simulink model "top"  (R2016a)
settings: Solver=FixedStepAuto  StartTime=0.0  StopTime=0.1  RelTol=1e-3
PreLoadFcn:
  | % ---  DO NOT REMOVE THIS CODE (2025.1)   ---
  |     % create Simulink variants
  |     if not(exist('variant_simulation', 'var'))
  |         variant_simulation = Simulink.Variant('SIMULINK_MODE==0');
  |     end
  |     if not(exist('variant_generation', 'var'))
  |         variant_generation = Simulink.Variant('SIMULINK_MODE==1');
  |     end
  | 
  |     % check SDK version
  |     required_lib_version = 3900.3;
  |     required_lib_ver_str = '2025.1';
  |     lib_path = [getenv('IX_SIMULINK_ACG_BB_3') '\simulink\blocks\BoomBox.slx'];
  |     if exist(lib_path, 'file')
  |         lib_version = str2double(Simulink.MDLInfo(lib_path).ModelVersion); % fullpath to avoid getting shadowing files
  |         if lib_version < required_lib_version || isnan(lib_version)
  |             error(['The model ''' bdroot ''' has been saved with a more recent version of ACG SDK (' required_lib_ver_str ') and might not work as expected. <a href="matlab:private_end_string = ''--- PLACE YOUR CODE BELOW THIS LINE ---'';private_fcn = get_param(bdroot, ''PreLoadFcn'');private_end_index = strfind(private_fcn, private_end_string);set_param(bdroot, ''PreLoadFcn'', strtrim(private_fcn(private_end_index(end)+length(private_end_string):end)));private_fcn = get_param(bdroot, ''PostLoadFcn'');private_end_index = strfind(private_fcn, private_end_string);set_param(bdroot, ''PostLoadFcn'', strtrim(private_fcn(private_end_index(end)+length(private_end_string):end)));private_fcn = get_param(bdroot, ''InitFcn'');private_end_index = strfind(private_fcn, private_end_string);set_param(bdroot, ''InitFcn'', strtrim(private_fcn(private_end_index(end)+length(private_end_string):end)));clear private_end_string private_fcn private_end_index;open(bdroot);">Click here</a> to continue anyway, or download the latest version of the SDK at <a href="www.imperix.com/downloads">www.imperix.ch/downloads</a>.']);
  |         end
  |     elseif exist(getenv('IX_SIMULINK_ACG_BB_3'), 'dir')
  |         error(['Library file for imperix ACG SDK not found in path ''' lib_path '''. Please try to re-install ACG SDK (<a href="www.imperix.com/downloads">www.imperix.ch/downloads</a>).']);
  |     else
  |         error('ACG SDK is not installed on this computer and the model will not work as expected. Please download ACG SDK at <a href="www.imperix.com/downloads">www.imperix.ch/downloads</a>, install it, and reopen the model.');
  |     end
  |     clear required_lib_version required_lib_ver_str lib_path lib_version;
  | 
  |     ix_acg_path = getenv('IX_SIMULINK_ACG_BB_3');
  |     addpath(fullfile(ix_acg_path, 'simulink\target'));
  |     addpath(fullfile(ix_acg_path, 'simulink\blocks'));
  |     addpath(fullfile(ix_acg_path, 'simulink\functions'));
  |     sl_refresh_customizations;
  |     clear ix_acg_path;
  | 
  |     % The SIMULINK_MODE variable is created in the base
  |     % workspace in the PostLoadFcn from the block whose id is kb0101
  |     % All opened models share a common variant configuration.
  | 
  |     Model_PreLoadFcn(bdroot);
  | % --- PLACE YOUR CODE BELOW THIS LINE ---
PostLoadFcn:
  | % ---  DO NOT REMOVE THIS CODE (2025.1)   ---
  |     % change the execution mode of simulink depending on the radio button:
  |     if(strcmp('Automated Code Generation',get_param(Find_imperix_blocks(bdroot,'Configuration'),'SLMODE')))
  |         assignin('base', 'SIMULINK_MODE', 1);
  |     else
  |         assignin('base', 'SIMULINK_MODE', 0);
  |     end
  | 
  |     Model_PostLoadFcn(bdroot);
  | % --- PLACE YOUR CODE BELOW THIS LINE ---
InitFcn:
  | % ---  DO NOT REMOVE THIS CODE (2025.1)   ---
  |     % check SDK version
  |     required_lib_version = 3900.3;
  |     required_lib_ver_str = '2025.1';
  |     lib_path = [getenv('IX_SIMULINK_ACG_BB_3') '\simulink\blocks\BoomBox.slx'];
  |     if exist(lib_path, 'file')
  |         lib_version = str2double(Simulink.MDLInfo(lib_path).ModelVersion); % fullpath to avoid getting shadowing files
  |         if lib_version < required_lib_version || isnan(lib_version)
  |             error(['The model ''' bdroot ''' has been saved with a more recent version of ACG SDK (' required_lib_ver_str ') and might not work as expected. <a href="matlab:private_end_string = ''--- PLACE YOUR CODE BELOW THIS LINE ---'';private_fcn = get_param(bdroot, ''PreLoadFcn'');private_end_index = strfind(private_fcn, private_end_string);set_param(bdroot, ''PreLoadFcn'', strtrim(private_fcn(private_end_index(end)+length(private_end_string):end)));private_fcn = get_param(bdroot, ''PostLoadFcn'');private_end_index = strfind(private_fcn, private_end_string);set_param(bdroot, ''PostLoadFcn'', strtrim(private_fcn(private_end_index(end)+length(private_end_string):end)));private_fcn = get_param(bdroot, ''InitFcn'');private_end_index = strfind(private_fcn, private_end_string);set_param(bdroot, ''InitFcn'', strtrim(private_fcn(private_end_index(end)+length(private_end_string):end)));clear private_end_string private_fcn private_end_index;open(bdroot);">Click here</a> to continue anyway, or download the latest version of the SDK at <a href="www.imperix.com/downloads">www.imperix.ch/downloads</a>.']);
  |         end
  |     elseif exist(getenv('IX_SIMULINK_ACG_BB_3'), 'dir')
  |         error(['Library file for imperix ACG SDK not found in path ''' lib_path '''. Please try to re-install ACG SDK (<a href="www.imperix.com/downloads">www.imperix.ch/downloads</a>).']);
  |     else
  |         error('ACG SDK is not installed on this computer and the model will not work as expected. Please download ACG SDK at <a href="www.imperix.com/downloads">www.imperix.ch/downloads</a>, install it, and reopen the model.');
  |     end
  |     clear required_lib_version required_lib_ver_str lib_path lib_version;
  | 
  |     Model_InitFcn(bdroot);
  | % --- PLACE YOUR CODE BELOW THIS LINE ---
model workspace (MAT data in the model file):
  TSAMPLE = 2e-06
  global_CLK_number = 0
  global_INT_number = 1
  global_SVM_instance_id = 0
  global_comp_time = 0.2
undefined symbols (not defined in the file): Configuration_InitFcn

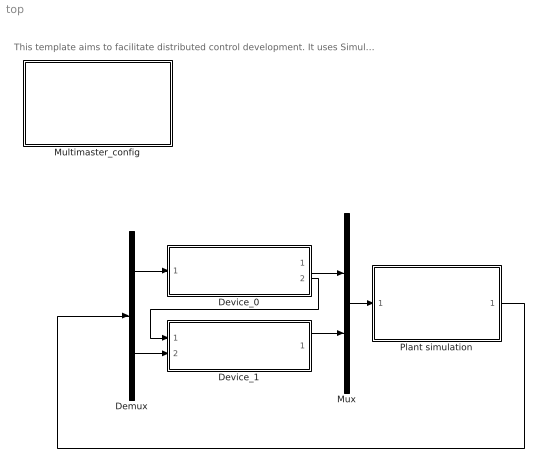
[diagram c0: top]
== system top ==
  note: This template aims to facilitate distributed control development. It uses Simulink model references to support both simulation and code generation in the same development environment. Requires imperix ACG SDK 2025.1 or more recent. To learn more, please visite the following knowledge base page: https://imperix.com/doc/help/multi-master-mode-for-distributed-networked-control-systems
  Demux : Demux  Outputs=2
  Device_0 : ModelReference  ModelNameDialog=model_a  SimulationMode=Normal  ModelReferenceVersion=1.108
  Device_1 : ModelReference  ModelNameDialog=model_b  SimulationMode=Normal  ModelReferenceVersion=1.103
  Multimaster_config : Subsystem  Description=Please leave the Priority (below parameter) to maximum negative to ensure that this block is always executed first.  Priority=-99999  InitFcn=Configuration_InitFcn(bdroot);
  Mux : Mux  Inputs=2
  Plant simulation : Subsystem
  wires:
  Device_0/1 -> Mux/1
  Device_1/1 -> Mux/2
  Demux/1 -> Device_0/1
  Mux/1 -> Plant simulation/1(Inputs)
  Plant simulation/1(Outputs) -> Demux/1
  Demux/2 -> Device_1/2
  Device_0/2 -> Device_1/1

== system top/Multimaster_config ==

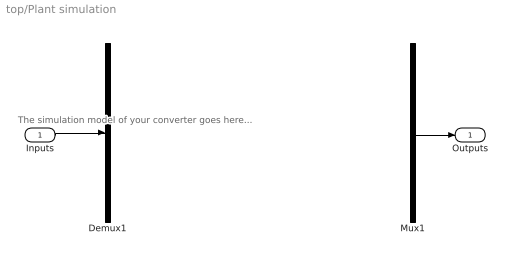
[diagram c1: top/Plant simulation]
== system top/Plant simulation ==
  note: The simulation model of your converter goes here...
  Inputs : Inport
  Demux1 : Demux  Outputs=10
  Mux1 : Mux  Inputs=10
  Outputs : Outport
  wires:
  Inputs/1 -> Demux1/1
  Mux1/1 -> Outputs/1
